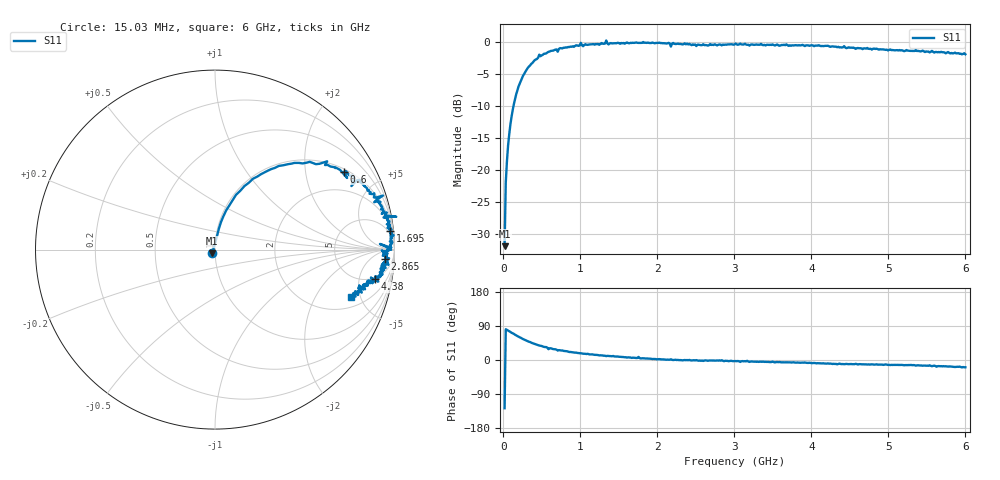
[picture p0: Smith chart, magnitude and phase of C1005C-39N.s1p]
!	Network	Analyzer	HP8753E.07.74:	Oct	30	2002	Serial	No.	JP38451487
!	Hewlett-Packard
!	7	Sep	2009	9:07:06
!	Frequency	S11
#	HZ	S	RI	R	50
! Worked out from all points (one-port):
!   400 points, 15.03 MHz to 6 GHz, reference 50 ohm
!   lowest |S11| = -31.8 dB at 15.03 MHz (marker M1), VSWR 1.05, Z = 48.4 - j1.98 ohm
!   |S11| at or under -10 dB: start of sweep to 130.4 MHz
!   S11 on the Smith chart (normalised r, x): 15.03 MHz: 0.97, -0.04; 600 MHz: 1.09, +3.25; 1.695 GHz: 3, +18; 2.865 GHz: 18, -19; 4.38 GHz: 4.53, -8.53; 6 GHz: 2.81, -4.10
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1.502992e7  -0.0155 -0.0204
3.002985e7  0.0122 0.0791
4.502978e7  0.0212 0.115
9.002955e7  0.0621 0.218
1.350293e8  0.117 0.305
3.150284e8  0.407 0.476
4.650277e8  0.625 0.492
6.00027e8  0.72 0.435
7.650262e8  0.806 0.378
1.005025e9  0.936 0.301
1.035025e9  0.887 0.264
1.320023e9  0.953 0.19
1.335023e9  1.01 0.183
1.365023e9  0.939 0.179
1.515022e9  0.957 0.141
1.695022e9  0.977 0.103
1.755021e9  0.972 0.139
1.785021e9  0.981 0.068
2.145019e9  0.983 0.0116
2.175019e9  0.919 0.0315
2.265019e9  0.97 0.00366
2.865016e9  0.947 -0.0537
3.015015e9  0.97 -0.0485
3.765011e9  0.933 -0.0985
4.380008e9  0.893 -0.165
4.515007e9  0.888 -0.165
5.265004e9  0.83 -0.198
6e9  0.757 -0.262
